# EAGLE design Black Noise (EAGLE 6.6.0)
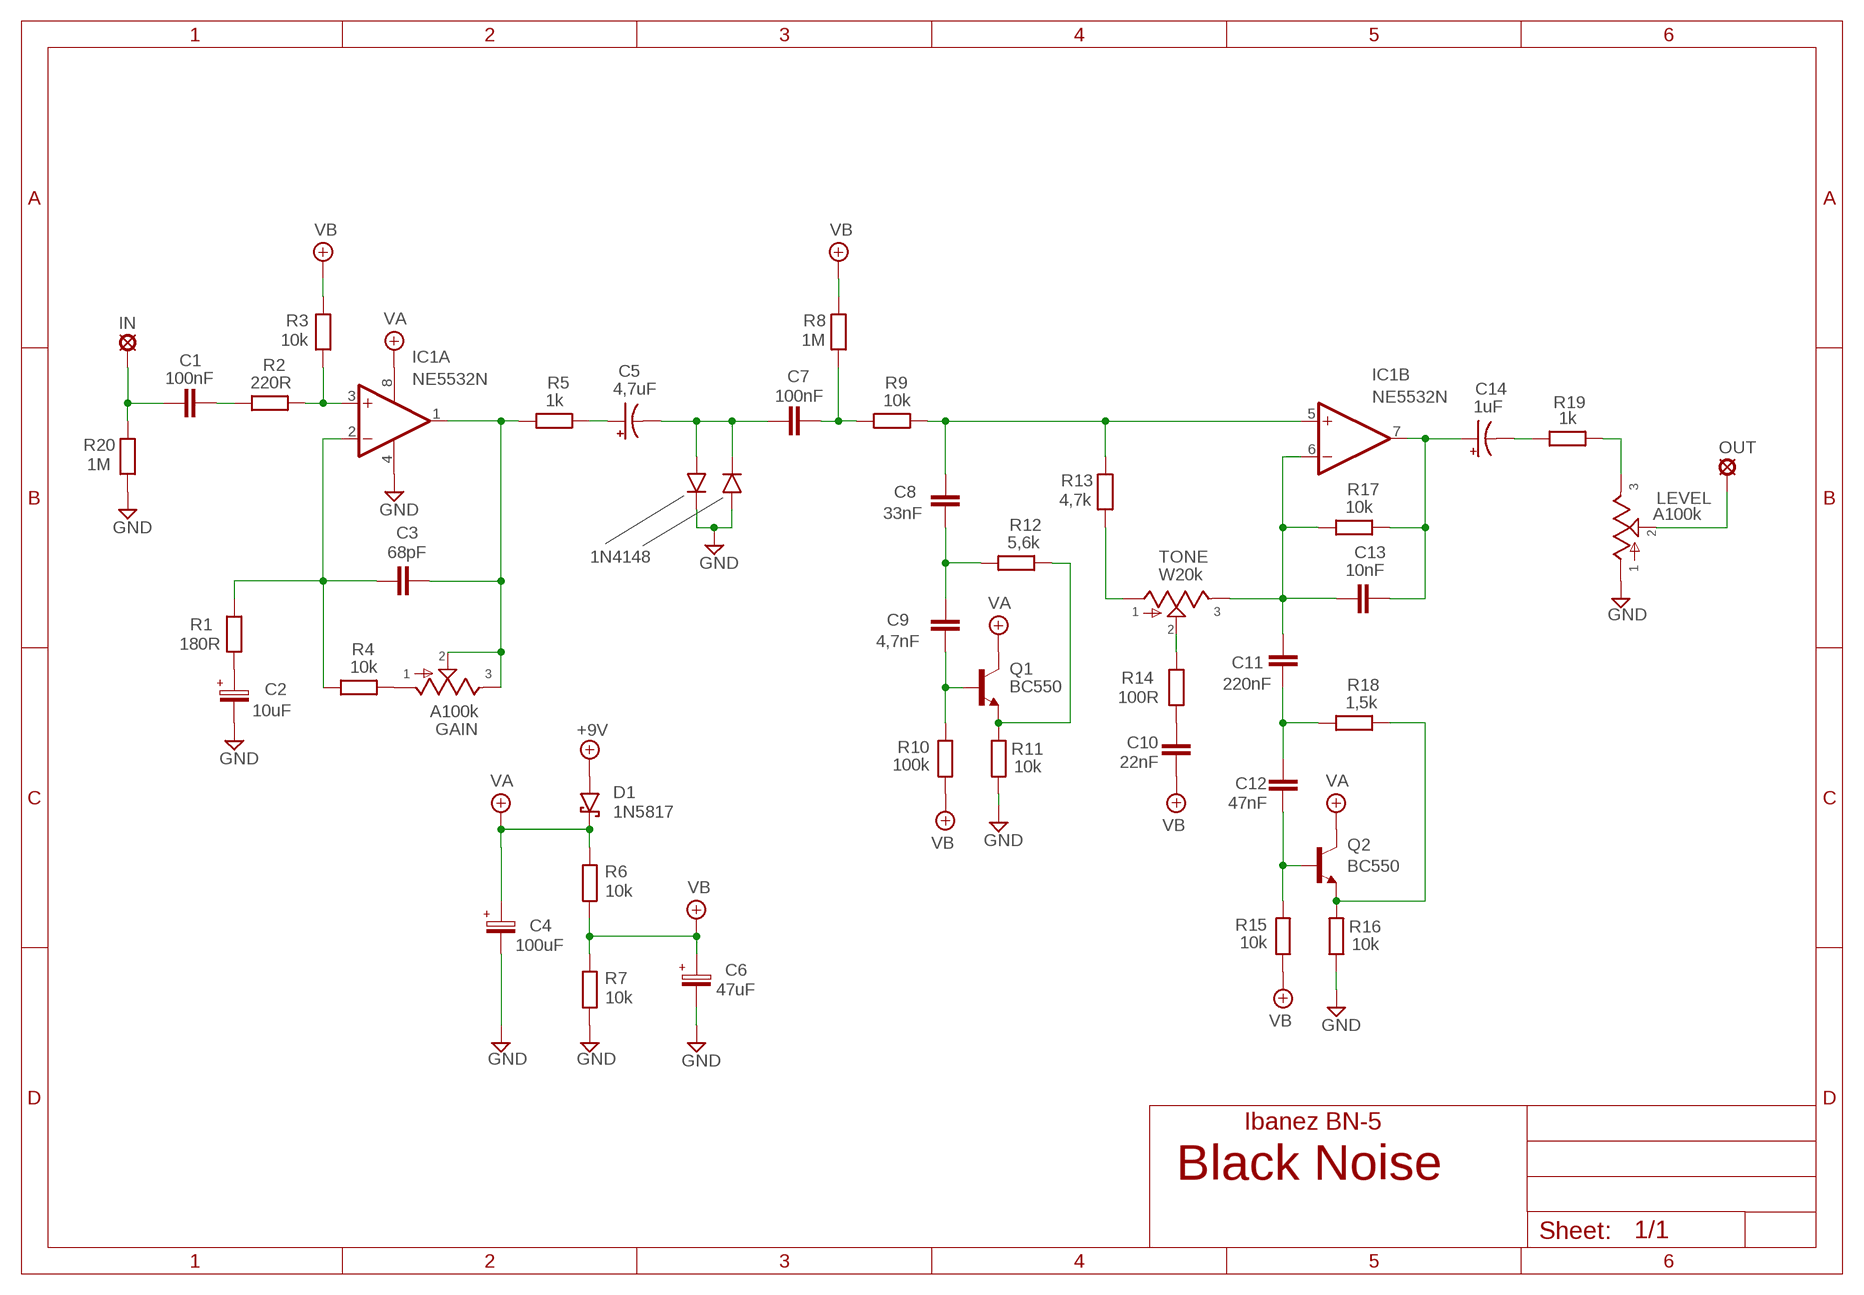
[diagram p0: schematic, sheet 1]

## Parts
+9V  +9V  +9V(T)1  [ROUND]
C1  100nF  100NF-220NF  [7,5MM]
C2  10uF  063-EU  [063_025]
C3  68pF  050X030_0252  [050X030_025_2]
C4  100uF  063-EU  [063_025]
C5  4,7uF  044A1  [044A]
C6  47uF  063-EU  [063_025]
C7  100nF  100NF-220NF  [7,5MM]
C8  33nF  22NF-82NF"  [4,5MM]
C9  4,7nF  1NF-15NF  [3,5MM]
C10  22nF  22NF-82NF"  [4,5MM]
C11  220nF  100NF-220NF  [7,5MM]
C12  47nF  22NF-82NF"  [4,5MM]
C13  10nF  1NF-15NF  [3,5MM]
C14  1uF  044A1  [044A]
D1  1N5817  [DO41-3]
D2  1N4148-3  [DO35-3]
D3  1N4148-3  [DO35-3]
GAIN  A100k  POT16MM  [16MM]
GND  GND  GND(T)1  [ROUND]
GND4  GND  GND(T)1  [ROUND]
IC1  NE5532N  [DIL08]
IN  MCS10B  [MCS10B]
LEVEL  A100k  POT16MM  [16MM]
OUT  MCS10B  [MCS10B]
Q1  BC550  [TO92-]
Q2  BC550  [TO92-]
R1  180R  6MM-EU3  [R0207/3]
R2  220R  6MM-EU3  [R0207/3]
R3  10k  6MM-EU3  [R0207/3]
R4  10k  6MM-EU3  [R0207/3]
R5  1k  6MM-EU3  [R0207/3]
R6  10k  6MM-EU3  [R0207/3]
R7  10k  6MM-EU3  [R0207/3]
R8  1M  6MM-EU3  [R0207/3]
R9  10k  6MM-EU3  [R0207/3]
R10  100k  6MM-EU3  [R0207/3]
R11  10k  6MM-EU3  [R0207/3]
R12  5,6k  6MM-EU3  [R0207/3]
R13  4,7k  6MM-EU3  [R0207/3]
R14  100R  6MM-EU3  [R0207/3]
R15  10k  6MM-EU3  [R0207/3]
R16  10k  6MM-EU3  [R0207/3]
R17  10k  6MM-EU3  [R0207/3]
R18  1,5k  6MM-EU3  [R0207/3]
R19  1k  6MM-EU3  [R0207/3]
R20  1M  6MM-EU3  [R0207/3]
TONE  W20k  POT16MM  [16MM]

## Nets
+9V: +9V.1(+9V) D1.A
GND: C2.- C4.- C6.- D2.C D3.A GND4.1(GND) GND.1(GND) IC1.4(P:V-) LEVEL.1 R7.1 R11.1 R16.1 R20.1
N$1: C3.2 GAIN.2 GAIN.3 IC1.1(A:OUT) R5.1
N$2: C1.P$2 R2.1
N$3: C3.1 IC1.2(A:-IN) R1.2 R4.1
N$4: IC1.3(A:+IN) R2.2 R3.1
N$5: C1.P$1 IN.MP R20.2
N$6: GAIN.1 R4.2
N$7: C2.+ R1.1
N$8: C5.1(+) R5.2
N$9: C5.2(-) C7.P$1 D2.A D3.C
N$10: C7.P$2 R8.1 R9.1
N$11: C8.2 C9.1 R12.1
N$12: C9.2 Q1.2(B) R10.2
N$13: Q1.1(E) R11.2 R12.2
N$14: Q2.1(E) R16.2 R18.2
N$15: C11.P$1 C12.1 R18.1
N$16: C12.2 Q2.2(B) R15.2
N$17: C11.P$2 C13.1 IC1.6(B:-IN) R17.1 TONE.3
N$18: C13.2 C14.1(+) IC1.7(B:OUT) R17.2
N$19: R13.1 TONE.1
N$20: R14.2 TONE.2
N$21: C10.1 R14.1
N$22: C8.1 IC1.5(B:+IN) R9.2 R13.2
N$23: C14.2(-) R19.1
N$24: LEVEL.3 R19.2
N$25: LEVEL.2 OUT.MP
VA: C4.+ D1.C IC1.8(P:V+) Q1.3(C) Q2.3(C) R6.2
VB: C6.+ C10.2 R3.2 R6.1 R7.2 R8.2 R10.1 R15.1

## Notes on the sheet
- 1N4148
- Ibanez BN-5

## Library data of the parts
+9V = gm-supply:+9V(T): +9V Voltage Supply
C1 C7 C11 = Mylar Kondensaattorit:100NF-220NF: 100nF-220nF
C2 C4 C6 = Elektrolyytit:063-EU
C3 = Keraamiset kondensaattorit:050X030_025: 47 - 120pF
C5 C14 = Tantaalit:044A: .1 - 1.5µF
C8 C10 C12 = Mylar Kondensaattorit:22NF-82NF: 22nF-82nF
C9 C13 = Mylar Kondensaattorit:1NF-15NF: 1nF-15nF
D1 = Diodit:1N5817
D2 D3 = Diodit:1N4148: Fast Switching Diode
GAIN LEVEL TONE = gm-pots:POT: Potentiometers the arrow indicates the clockwise motion of th wiper (lug 2) fully counter clockwise there is no resistance between lugs 1 and 2 fully clockwise the resistance between lugs 1 and 2 is the value of the pot
GND GND4 = gm-supply:GND(T): Ground
IC1 = Operaatiovahvistimet:NE5532: AUDIO AMPLIFIER
IN OUT = Padit:MCS10B: SOLDER PAD
Q1 Q2 = Transistorit:BC550
R1-R20 = Vastukset:6MM-EU: 6mm Resistors (European schematic symbol)

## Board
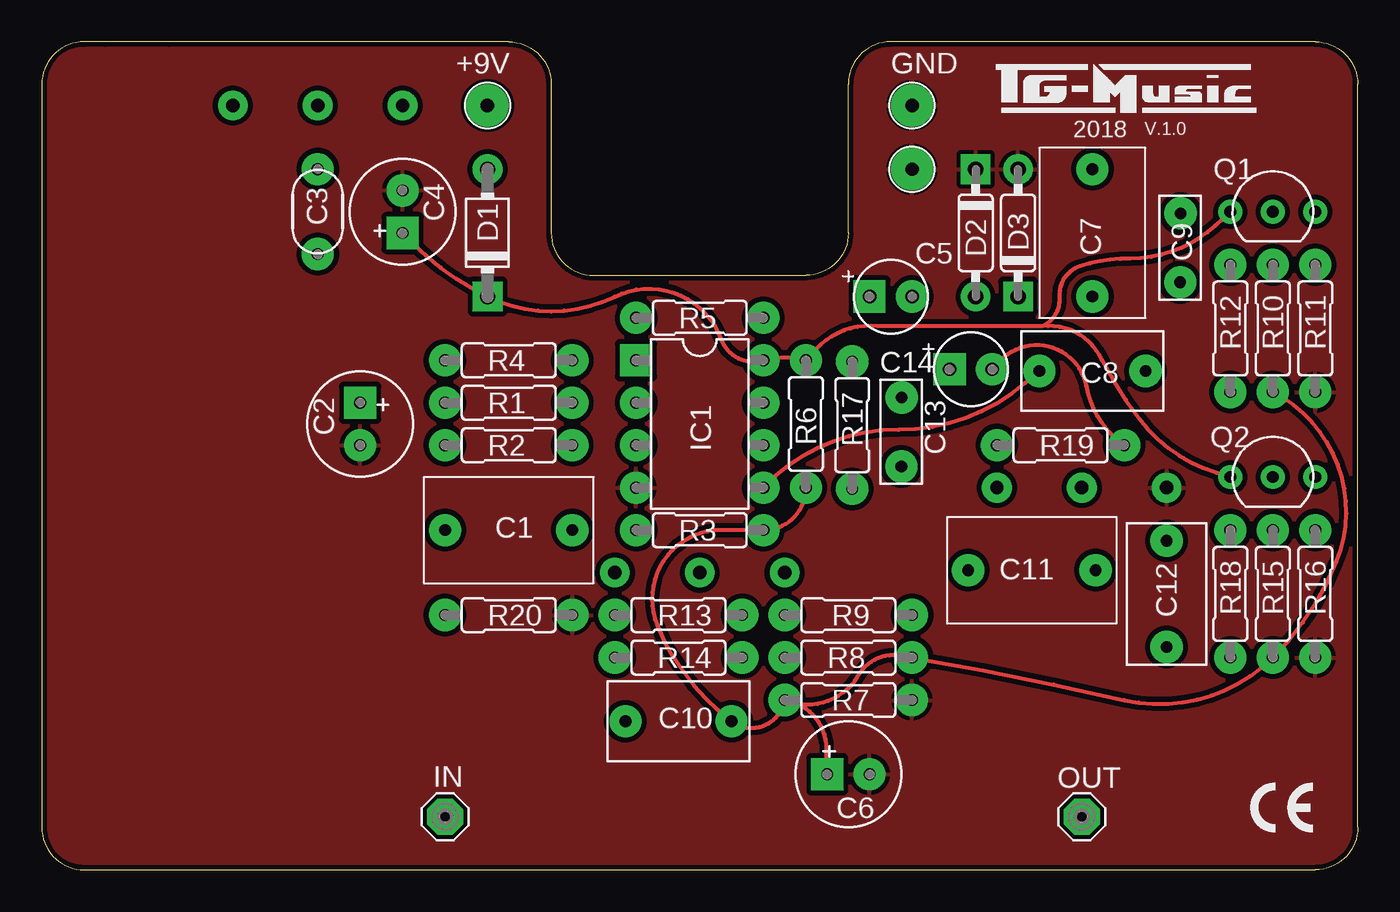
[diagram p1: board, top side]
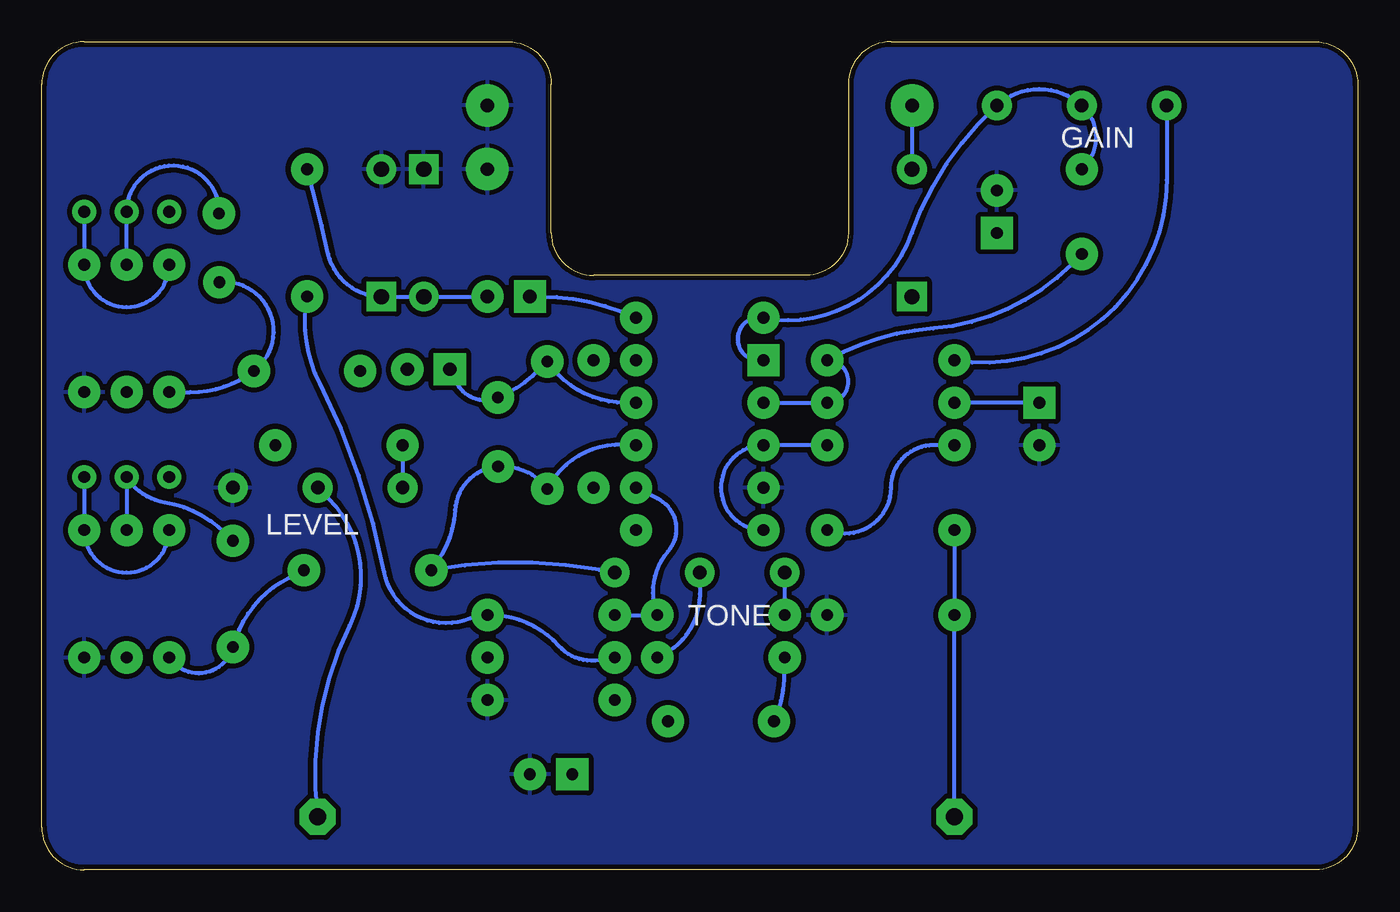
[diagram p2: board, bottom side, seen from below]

Size 78.74 x 49.53 mm. Coordinates in mm from the lower left corner, seen from the top.
Outline: 7.62,49.53 3.81,49.53
Outline: 78.74,2.54 78.74,46.99 arc90 76.2,49.53 50.8,49.53 arc90 48.26,46.99 48.26,38.1 arc-90 45.72,35.56 33.02,35.56 arc-90 30.48,38.1 30.48,46.99 arc90 27.94,49.53 2.54,49.53 arc90 0,46.99 0,2.54 arc90 2.54,0 76.2,0 arc90 78.74,2.54
Copper layers (1*16): Top 0.035mm / dielectric 1.5mm / Bottom 0.035mm
Design rules "ITEADstudio": minimum track width 10mil, minimum drill 12mil, track to track 12mil, track to pad 12mil, pad to pad 12mil, via to via 12mil, smd to smd 0mil, copper to edge 12mil, drill to drill 12mil, minimum pad ring 10mil, minimum via ring 6mil, stop-mask expansion 4mil, vias tented up to drill 100mil, thermal gap 10mil

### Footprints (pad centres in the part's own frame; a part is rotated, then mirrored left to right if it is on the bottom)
ROUND = drill 0.8 pad 2.54: 1 0,0
7,5MM = drill 0.7 pad 1.93: P$1 -3.81,0; P$2 3.81,0
063_025 = drill 0.7 pad 1.93 square: + -1.27,0 | drill 0.7 pad 1.93: - 1.27,0
050X030_025_2 = drill 0.7 pad 1.93: 1 -2.54,0; 2 2.54,0
044A = drill 0.8 pad 1.93 square: 1 -1.27,0 | drill 0.8 pad 1.93: 2 1.27,0
4,5MM = drill 0.7 pad 1.93: 1 -3.175,0; 2 3.175,0
3,5MM = drill 0.7 pad 1.93: 1 -1.905,0; 2 2.221,-0.016
DO41-3 = drill 0.9 pad 1.778: A 3.81,0 | drill 0.9 pad 1.778 square: C -3.81,0
DO35-3 = drill 0.9 pad 1.778: A 3.81,0 | drill 0.9 pad 1.778 square: C -3.81,0
16MM = drill 0.8 pad 1.778: 1 5.08,0; 2 0,0; 3 -5.08,0
DIL08 = drill 0.7 pad 1.93 square: 1 -3.81,-3.81 | drill 0.7 pad 1.93: 2 -1.27,-3.81; 3 1.27,-3.81; 4 3.81,-3.81; 5 3.81,3.81; 6 1.27,3.81; 7 -1.27,3.81; 8 -3.81,3.81
MCS10B = drill 1.016 pad 2.159 octagon: MP 0,0
TO92- = drill 0.7 pad 1.422: 1 2.54,0; 2 0,0; 3 -2.54,0
R0207/3 = drill 0.7 pad 1.93: 1 -3.81,0; 2 3.81,0

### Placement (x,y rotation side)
+9V  26.67,45.72 0 top
C1  27.94,20.32 0 top
C2  19.05,26.67 270 top
C3  16.51,39.37 90 top
C4  21.59,39.37 90 top
C5  50.8,34.29 0 top
C6  48.26,5.71 0 top
C7  62.87,38.1 270 top
C8  62.87,29.84 0 top
C9  68.12,37.05 90 top
C10  38.1,8.89 0 top
C11  59.24,17.92 180 top
C12  67.31,16.51 90 top
C13  51.44,26.04 90 top
C14  55.6,29.94 0 top
D1  26.67,38.1 90 top
D2  55.88,38.1 270 top
D3  58.42,38.1 90 top
GAIN  16.51,45.72 0 bottom
GND  52.07,45.72 0 top
GND4  52.07,41.91 0 top
IC1  39.37,26.67 270 top
IN  24.13,3.17 0 top
LEVEL  62.23,22.86 180 bottom
OUT  62.23,3.17 0 top
Q1  73.66,39.37 0 top
Q2  73.66,23.5 0 top
R1  27.94,27.94 0 top
R2  27.94,25.4 0 top
R3  39.37,20.32 0 top
R4  27.94,30.48 180 top
R5  39.37,33.02 0 top
R6  45.72,26.67 90 top
R7  48.26,10.16 180 top
R8  48.26,12.7 0 top
R9  48.26,15.24 180 top
R10  73.66,32.38 90 top
R11  76.2,32.38 90 top
R12  71.12,32.38 90 top
R13  38.1,15.24 0 top
R14  38.1,12.7 0 top
R15  73.66,16.51 90 top
R16  76.2,16.51 90 top
R17  48.49,26.6 90 top
R18  71.12,16.51 90 top
R19  60.96,25.4 180 top
R20  27.94,15.24 180 top
TONE  39.37,17.78 0 bottom

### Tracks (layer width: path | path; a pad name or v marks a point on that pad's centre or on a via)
+9V
  Bottom 0.254: +9V.1 D1.A
GND
  pour Bottom: 0,2.54 0,46.99 arc-90 2.54,49.53 27.94,49.53 arc-90 30.48,46.99 30.48,38.1 arc90 33.02,35.56 45.72,35.56 arc90 48.26,38.1 48.26,46.99 arc-90 50.8,49.53 76.2,49.53 arc-90 78.74,46.99 78.74,2.54 arc-90 76.2,0 2.54,0 arc-90
  pour Top: 0,2.54 0,46.99 arc-90 2.54,49.53 27.94,49.53 arc-90 30.48,46.99 30.48,38.1 arc90 33.02,35.56 45.72,35.56 arc90 48.26,38.1 48.26,46.99 arc-90 50.8,49.53 76.2,49.53 arc-90 78.74,46.99 78.74,2.54 arc-90 76.2,0 2.54,0 arc-90
N$1
  Bottom 0.254: C3.2 arc-96 GAIN.2 arc-84 GAIN.3 arc-28 26.67,38.1 arc81 R5.1 arc-202 IC1.1
N$2
  Bottom 0.254: R2.1 25.4,25.4 arc-90 27.94,22.86 arc113 C1.P$2
N$3
  Bottom 0.254: IC1.2 R1.2 arc-180 R4.1 arc24 25.4,32.38 arc-40 17.14,36.2 C3.1
N$4
  Bottom 0.254: R2.2 IC1.3 arc-180 R3.1
N$5
  Bottom 0.254: C1.P$1 R20.2 IN.MP
N$6
  Bottom 0.254: GAIN.1 11.43,41.27 arc99 R4.2
N$7
  Bottom 0.254: C2.+ R1.1
N$8
  Bottom 0.254: C5.1 48.9,34.29 arc25 R5.2
N$9
  Bottom 0.254: C5.2 D2.A D3.C arc77 61.59,36.83 arc-3 C7.P$1
N$10
  Bottom 0.254: R8.1 45.37,12.54 arc57 47.79,13.39 arc-49 R9.1 arc-21 53.13,15.03 arc101 58.25,17.82 arc-16 62.09,29.08 arc37 C7.P$2
N$11
  Bottom 0.254: R12.1 69.85,28.57 arc-37 C8.2 arc-149 C9.1
N$12
  Bottom 0.254: R10.2 Q1.2 arc182 C9.2
N$13
  Bottom 0.254: Q1.1 R11.2 arc-180 R12.2
N$14
  Bottom 0.254: Q2.1 R16.2 arc-180 R18.2
N$15
  Bottom 0.254: C11.P$1 63.95,17.47 arc-48 C12.1 arc131 R18.1
N$16
  Bottom 0.254: R15.2 Q2.2 arc-49 71.37,21.97 arc36 67.72,20.09 C12.2
N$17
  Bottom 0.254: IC1.6 43.98,25.43 arc-65 R17.1 arc-58 C13.1 arc-82 54.02,21.52 arc35 C11.P$2 arc21 45.38,17.95 TONE.3
N$18
  Bottom 0.254: IC1.7 43.81,27.94 arc56 R17.2 arc26 C13.2 arc87 53.98,29.21 C14.1
N$19
  Bottom 0.254: TONE.1 R13.1
N$20
  Bottom 0.254: TONE.2 39.37,16.51 arc67 R14.2
N$21
  Bottom 0.254: R14.1 34.29,12.06 arc23 C10.1
N$22
  Top 0.254: C8.1 58.79,29.08 arc-41 51.27,26.32 arc47 IC1.5
  Bottom 0.254: IC1.5 41.91,22.23 arc104 41.27,19.05 arc-63 R13.2 R9.2
N$23
  Top 0.254: C14.2 57.35,30.46 arc-126 62.49,28.94 arc45 R19.1
N$24
  Bottom 0.254: R19.2 LEVEL.3
N$25
  Bottom 0.254: LEVEL.2 61.59,22.23 arc71 60.33,14.61 arc-33 OUT.MP
VA
  Top 0.254: C4.+ 22.23,37.47 arc19 D1.C arc52 34.29,34.29 arc-96 40.64,31.75 arc86 IC1.8 arc-33 R6.2 46.07,30.83 arc-59 50.01,32.52 59.89,32.52 | 59.89,32.52 arc-72 63.42,30.5 arc9 65.69,26.96 arc36 70.28,23.75 Q2.3 | Q1.3 70.22,38.53 arc-43 65.12,36.57 arc18 62.13,36.11 arc76 60.9,34.27 arc-67 59.89,32.52
VB
  Top 0.254: R6.1 arc-90 R3.2 40.64,20.32 arc113 36.83,14.61 arc31 C10.2 arc117 R7.2 | R7.2 arc83 48.83,11.6 arc-69 51.43,12.81 R8.2 arc-3 64.77,10.16 arc58 R15.1 arc23 77.47,18.41 arc85 R10.1 | C6.+ 46.96,7.27 arc80 R7.2

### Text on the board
tNames: 2018 | V.1.0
